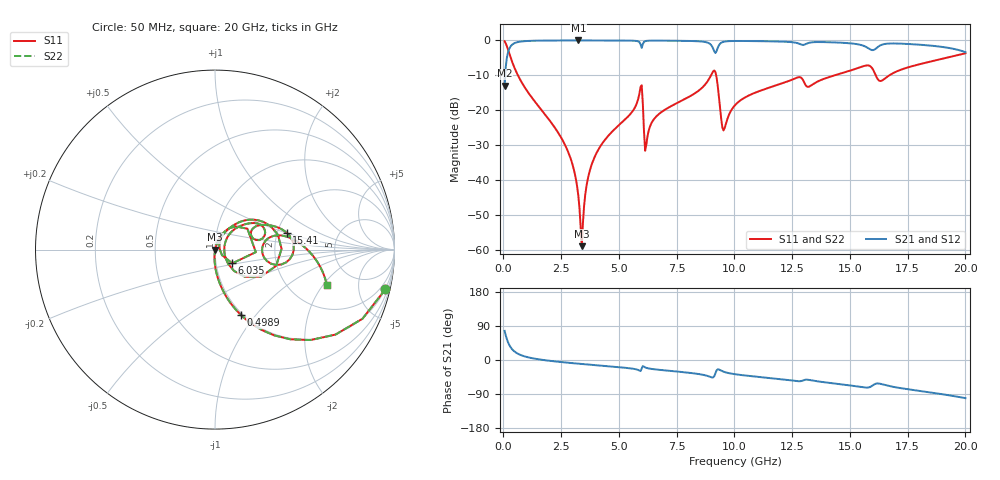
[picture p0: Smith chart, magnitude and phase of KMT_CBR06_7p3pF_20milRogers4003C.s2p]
! Data measured by Modelithics Inc. support@modelithics.com 813-866-6335
! KEMET CBR0603 7.3pF, Pad Width= 0.851mm, Pad Length= 0.64mm, Pad Gap= 0.62mm, 20mil Rogers 4003C substrate Data, January 2022
# hz S ma R 50
! 2 Port Network Data from SP1.SP block
! freq  magS11  angS11  magS21  angS21  magS12  angS12  magS22  angS22
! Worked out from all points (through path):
!   401 points, 50 MHz to 20 GHz, reference 50 ohm
!   highest |S21| = -0.01 dB at 3.242 GHz (marker M1); lowest = -12.9 dB at 50 MHz (marker M2)
!   group delay of S21, straight-line fit = 14.6 ps
!   lowest |S11| = -58.9 dB at 3.392 GHz (marker M3), VSWR 1.00, Z = 50.1 - j0.00212 ohm
!   |S11| at or under -10 dB: 627.2 MHz to 8.985 GHz (8.358 GHz wide, 174 % of centre); 9.209 GHz to 14.34 GHz (5.128 GHz wide, 43.6 % of centre); 16.12 GHz to 16.71 GHz (586.3 MHz wide, 3.57 % of centre)
!   |S22| runs from -58.9 to -0.2 dB; largest |S21 - S12| = 0
!   S11 on the Smith chart (normalised r, x): 50 MHz: 0.98, -8.54; 498.9 MHz: 0.98, -0.84; 6.035 GHz: 1.20, -0.19; 15.41 GHz: 2.24, +0.51; 20 GHz: 3.15, -2.20
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5e7  0.9742 -13.2  0.2254 76.8  0.2254 76.8  0.9742 -13.2
2.495e8  0.6525 -50.0  0.7572 40.0  0.7572 40.0  0.6525 -50.0
4.98875e8  0.3904 -68.5  0.92 21.4  0.92 21.4  0.3904 -68.5
2.6435e9  0.03304 -94.6  0.9984 -6.3  0.9984 -6.3  0.03304 -94.6
3.0425e9  0.0144 -94.4  0.9987 -8.6  0.9987 -8.6  0.0144 -94.4
3.242e9  0.005991 -89.2  0.9988 -9.7  0.9988 -9.7  0.005991 -89.2
3.391625e9  0.001136 -1.1  0.9988 -10.5  0.9988 -10.5  0.001136 -1.1
3.690875e9  0.01187 72.2  0.9986 -12.1  0.9986 -12.1  0.01187 72.2
4.089875e9  0.02666 73.1  0.9982 -14.2  0.9982 -14.2  0.02666 73.1
5.885375e9  0.1725 48.5  0.9448 -27.8  0.9448 -27.8  0.1725 48.5
6.035e9  0.1231 -38.4  0.8849 -15.9  0.8849 -15.9  0.1231 -38.4
6.184625e9  0.03208 41.2  0.9843 -20.7  0.9843 -20.7  0.03208 41.2
6.73325e9  0.08855 62.2  0.9928 -25.9  0.9928 -25.9  0.08855 62.2
9.077375e9  0.36 13.4  0.7667 -45.9  0.7667 -45.9  0.36 13.4
9.52625e9  0.05155 0.3  0.9552 -30.8  0.9552 -30.8  0.05155 0.3
1.0025e10  0.1184 47.0  0.9814 -37.5  0.9814 -37.5  0.1184 47.0
1.271825e10  0.2938 26.5  0.9164 -55.7  0.9164 -55.7  0.2938 26.5
1.336662e10  0.2325 28.1  0.9407 -54.0  0.9407 -54.0  0.2325 28.1
1.54115e10  0.4096 13.4  0.871 -70.8  0.871 -70.8  0.4096 13.4
1.605988e10  0.35 -14.2  0.7381 -64.2  0.7381 -64.2  0.35 -14.2
1.670825e10  0.3166 12.7  0.9026 -68.8  0.9026 -68.8  0.3166 12.7
2e10  0.6544 -17.7  0.6787 -100.6  0.6787 -100.6  0.6544 -17.7
